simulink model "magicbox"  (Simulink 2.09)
settings: Solver=ode1  StartTime=0.0  StopTime=1  FixedStep=0.001  MaxStep=0.001  RelTol=1e-5  AbsTol=1e-6

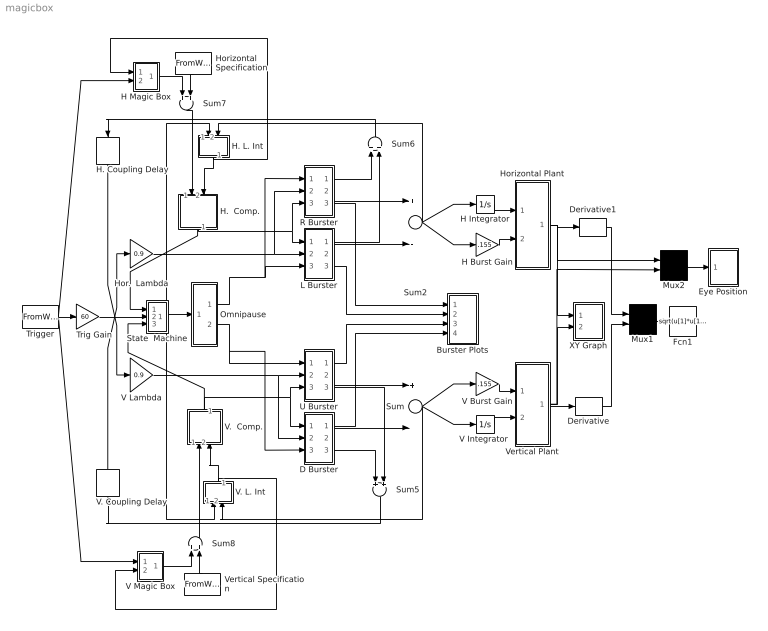
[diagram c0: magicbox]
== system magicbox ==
  Burster Plots : Subsystem
  D Burster : Subsystem
  Derivative : Derivative
  Derivative1 : Derivative
  Eye Position : Subsystem  mask(Graph scope.){}
      mask help: Graph scope using MATLAB graph window. Enter plotting ranges and line type.
      mask init:
      | color = @4; ax = [0, @1, @2, @3]; dt = -1;
  Fcn1 : Fcn  Expr=sqrt(u[1]*u[1]+u[2]*u[2])
  H Burst Gain : Gain  Gain=.155
  H Integrator : Integrator  ExternalReset=none  InitialConditionSource=internal  InitialCondition=0  LimitOutput=off  UpperSaturationLimit=inf  LowerSaturationLimit=-inf  ShowSaturationPort=off  ShowStatePort=off  AbsoluteTolerance=auto
  H Magic Box : Subsystem
  H.  Comp. : Subsystem  Orientation=down
  H. Coupling Delay : TransportDelay  Orientation=down  DelayTime=.001  InitialInput=00  BufferSize=1024
  H. L. Int : Subsystem  Orientation=down
  Hor.  Lambda : Gain  Gain=0.9
  Horizontal Plant : Subsystem
  "Horizontal Specification " : FromWorkspace  Orientation=down  VariableName=hspec
  L Burster : Subsystem
  Mux1 : Mux  Inputs=2
  Mux2 : Mux  Inputs=2
  Omnipause : Subsystem
  R Burster : Subsystem
  State  Machine : Subsystem
  Sum : Sum  Inputs=+-
  Sum2 : Sum  Inputs=+-
  Sum5 : Sum  Orientation=down  Inputs=++
  Sum6 : Sum  Orientation=up  Inputs=++
  Sum7 : Sum  Orientation=down  Inputs=++
  Sum8 : Sum  Orientation=up  Inputs=++
  Trig Gain : Gain  Gain=60
  Trigger : FromWorkspace  VariableName=trigspec
  U Burster : Subsystem
  V Burst Gain : Gain  Gain=.155
  "V Integrator " : Integrator  ExternalReset=none  InitialConditionSource=internal  InitialCondition=0  LimitOutput=off  UpperSaturationLimit=inf  LowerSaturationLimit=-inf  ShowSaturationPort=off  ShowStatePort=off  AbsoluteTolerance=auto
  V Lambda : Gain  Gain=0.9
  V Magic Box : Subsystem
  V.  Comp. : Subsystem  Orientation=up
  V. Coupling Delay : TransportDelay  Orientation=up  DelayTime=.001  InitialInput=00  BufferSize=1024
  V. L. Int : Subsystem  Orientation=up
  Vertical Plant : Subsystem
  Vertical Specification : FromWorkspace  Orientation=up  VariableName=vspec
  XY Graph : Subsystem  mask(XY scope.){}
      mask help: XY scope using MATLAB graph window. First input is used as time base. Enter plotting ranges.
      mask init:
      | ax = [@1, @2, @3, @4];st=-1;
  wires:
  H Integrator/1 -> Horizontal Plant/1(in_1)
  H Burst Gain/1 -> Horizontal Plant/2(in_2)
  Sum2/1 -> H Integrator/1, H Burst Gain/1, H. L. Int/2(BURST Input)
  V Burst Gain/1 -> Vertical Plant/1(in_1)
  "V Integrator "/1 -> Vertical Plant/2(in_2)
  Sum/1 -> V Burst Gain/1, "V Integrator "/1, V. L. Int/2(BURST Input)
  L Burster/2(out_2) -> Sum2/2
  R Burster/2(out_3) -> Sum2/1
  U Burster/3(out_4) -> Sum5/2
  U Burster/2(out_3) -> Sum/1
  U Burster/1(out_2) -> Burster Plots/3(in_3)
  D Burster/3(out_3) -> Sum5/1
  D Burster/2(out_2) -> Sum/2
  D Burster/1(out_1) -> Burster Plots/4(in_4)
  L Burster/3(out_3) -> Burster Plots/2(in_2)
  R Burster/3(out_4) -> Burster Plots/1(in_1)
  V Lambda/1 -> U Burster/2(in_2), D Burster/2(in_2)
  L Burster/1(out_1) -> Sum6/2
  Sum6/1 -> H. Coupling Delay/1
  Sum5/1 -> V. Coupling Delay/1
  Vertical Plant/1(out_1) -> XY Graph/2(y), Derivative/1, Mux2/2
  Mux1/1 -> Fcn1/1
  Derivative/1 -> Mux1/2
  Derivative1/1 -> Mux1/1
  Fcn1/1 -> ?
  R Burster/1(out_2) -> Sum6/1
  V. Coupling Delay/1 -> Hor.  Lambda/1
  H. Coupling Delay/1 -> V Lambda/1
  Horizontal Plant/1(out_1) -> XY Graph/1(x), Derivative1/1, Mux2/1
  Mux2/1 -> Eye Position/1(x)
  Hor.  Lambda/1 -> L Burster/2(in_2), R Burster/2(in_2)
  Omnipause/1(out_1) -> L Burster/3(in_3), R Burster/1(in_3)
  Omnipause/2(out_4) -> D Burster/3(in_3), U Burster/1(in_3)
  H.  Comp./1(out_1) -> L Burster/1(in_1), R Burster/3(in_1), State  Machine/1(in_1)
  V.  Comp./1(out_1) -> U Burster/3(in_1), D Burster/1(in_1), State  Machine/3(in_3)
  Trig Gain/1 -> State  Machine/2(in_2)
  State  Machine/1(out_2) -> V. L. Int/1(OPN Input), Omnipause/1(in_1), H. L. Int/1(STATE Input)
  "Horizontal Specification "/1 -> Sum7/2
  H Magic Box/1(out_1) -> Sum7/1
  Sum7/1 -> H.  Comp./1(in_1)
  H. L. Int/1(out_1) -> H.  Comp./2(in_2), H Magic Box/1(Current Displacement)
  Sum8/1 -> V.  Comp./1(in_4)
  Vertical Specification/1 -> Sum8/2
  V Magic Box/1(out_1) -> Sum8/1
  Trigger/1 -> Trig Gain/1, H Magic Box/2(Snapshot Trigger), V Magic Box/1(Current Displacement)
  V. L. Int/1(out_1) -> V.  Comp./2(in_5), V Magic Box/2(Snapshot Trigger)

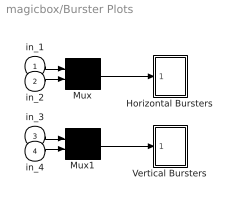
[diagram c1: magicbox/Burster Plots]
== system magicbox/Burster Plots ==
  in_1 : Inport  Port=1  PortWidth=-1  SampleTime=-1
  in_2 : Inport  Port=2  PortWidth=-1  SampleTime=-1
  in_3 : Inport  Port=3  PortWidth=-1  SampleTime=-1
  in_4 : Inport  Port=4  PortWidth=-1  SampleTime=-1
  Horizontal Bursters : Subsystem  mask(Graph scope.){}
      mask help: Graph scope using MATLAB graph window. Enter plotting ranges and line type.
      mask init:
      | color = @4; ax = [0, @1, @2, @3]; dt = -1;
  Mux : Mux  Inputs=2
  Mux1 : Mux  Inputs=2
  Vertical Bursters : Subsystem  mask(Graph scope.){}
      mask help: Graph scope using MATLAB graph window. Enter plotting ranges and line type.
      mask init:
      | color = @4; ax = [0, @1, @2, @3]; dt = -1;
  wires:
  Mux1/1 -> Vertical Bursters/1(x)
  Mux/1 -> Horizontal Bursters/1(x)
  in_1/1 -> Mux/1
  in_2/1 -> Mux/2
  in_3/1 -> Mux1/1
  in_4/1 -> Mux1/2

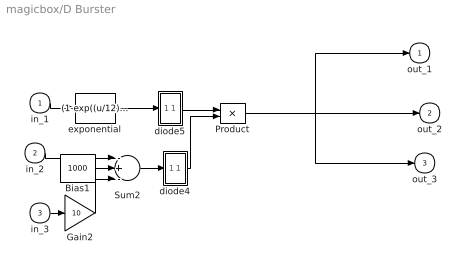
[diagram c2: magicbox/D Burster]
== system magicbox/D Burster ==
  in_1 : Inport  Port=1  PortWidth=-1  SampleTime=-1
  in_2 : Inport  Port=2  PortWidth=-1  SampleTime=-1
  in_3 : Inport  Port=3  PortWidth=-1  SampleTime=-1
  Bias1 : Constant  Value=1000
  Gain2 : Gain  Gain=10
  Product : Product  Inputs=2
  Sum2 : Sum  Inputs=-+-
  diode4 : Subsystem
  diode5 : Subsystem
  exponential : Fcn  Expr=(1-exp((u/12)))
  out_1 : Outport  Port=1  InitialOutput=0
  out_2 : Outport  Port=2  InitialOutput=0
  out_3 : Outport  Port=3  InitialOutput=0
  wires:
  Product/1 -> out_3/1, out_2/1, out_1/1
  diode5/1(out_1) -> Product/1
  exponential/1 -> diode5/1(in_1)
  diode4/1(out_1) -> Product/2
  Sum2/1 -> diode4/1(in_1)
  Gain2/1 -> Sum2/3
  in_3/1 -> Gain2/1
  in_2/1 -> Sum2/1
  Bias1/1 -> Sum2/2
  in_1/1 -> exponential/1

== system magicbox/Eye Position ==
  x : Inport  Port=1  PortWidth=-1  SampleTime=-1
  "S-function M-file which plots lines " : S-Function  FunctionName=sfuny  Parameters=ax, color,dt
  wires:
  x/1 -> "S-function M-file which plots lines "/1

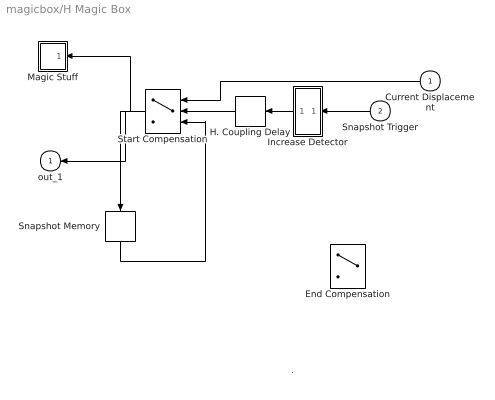
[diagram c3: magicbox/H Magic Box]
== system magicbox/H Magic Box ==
  note: .
  Current Displacement : Inport  Orientation=left  Port=1  PortWidth=-1  SampleTime=-1
  Snapshot Trigger : Inport  Orientation=left  Port=2  PortWidth=-1  SampleTime=-1
  " Snapshot Memory" : Memory  Orientation=down  X0=0  InheritSampleTime=off
  End Compensation : Switch  Orientation=left  Threshold=-2
  H. Coupling Delay : TransportDelay  Orientation=left  DelayTime=.002  InitialInput=00  BufferSize=1024
  Increase Detector : Subsystem  Orientation=left
  Magic Stuff : Subsystem  Orientation=left  mask(Graph scope.){}
      mask help: Graph scope using MATLAB graph window. Enter plotting ranges and line type.
      mask init:
      | color = @4; ax = [0, @1, @2, @3]; dt = -1;
  Start Compensation : Switch  Orientation=left  Threshold=0.001
  out_1 : Outport  Orientation=left  Port=1  InitialOutput=0
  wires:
  " Snapshot Memory"/1 -> Start Compensation/3
  Current Displacement/1 -> Start Compensation/1
  Start Compensation/1 -> " Snapshot Memory"/1, out_1/1, Magic Stuff/1(x)
  Snapshot Trigger/1 -> Increase Detector/1(Signal)
  Increase Detector/1(out_1) -> H. Coupling Delay/1
  H. Coupling Delay/1 -> Start Compensation/2

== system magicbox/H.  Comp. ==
  in_1 : Inport  Port=1  PortWidth=-1  SampleTime=-1
  in_2 : Inport  Port=2  PortWidth=-1  SampleTime=-1
  Sum : Sum  Inputs=+-
  out_1 : Outport  Port=1  InitialOutput=0
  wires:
  Sum/1 -> out_1/1
  in_1/1 -> Sum/1
  in_2/1 -> Sum/2

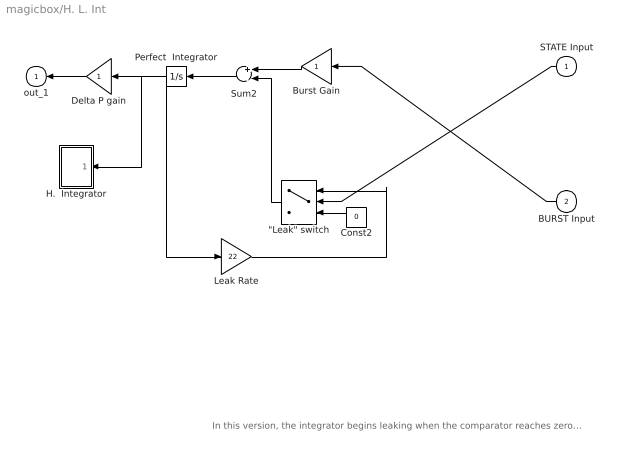
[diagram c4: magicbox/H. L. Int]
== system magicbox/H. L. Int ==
  note: In this version, the integrator begins leaking when the comparator reaches zero, and won't stop leaking until either the trigger arrives or the integrator's value goes to zero
  STATE Input : Inport  Orientation=left  Port=1  PortWidth=-1  SampleTime=-1
  BURST Input : Inport  Orientation=left  Port=2  PortWidth=-1  SampleTime=-1
  "\"Leak\" switch" : Switch  Orientation=left  Threshold=0.5
  Burst Gain : Gain  Orientation=left  Gain=1
  Const2 : Constant  Orientation=left  Value=0
  Delta P gain : Gain  Orientation=left  Gain=1
  H.  Integrator : Subsystem  Orientation=left  mask(Graph scope.){}
      mask help: Graph scope using MATLAB graph window. Enter plotting ranges and line type.
      mask init:
      | color = @4; ax = [0, @1, @2, @3]; dt = -1;
  Leak Rate : Gain  Gain=22
  Perfect  Integrator : Integrator  Orientation=left  ExternalReset=none  InitialConditionSource=internal  InitialCondition=0  LimitOutput=off  UpperSaturationLimit=inf  LowerSaturationLimit=-inf  ShowSaturationPort=off  ShowStatePort=off  AbsoluteTolerance=auto
  Sum2 : Sum  Orientation=left  Inputs=+-
  out_1 : Outport  Orientation=left  Port=1  InitialOutput=0
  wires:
  Sum2/1 -> Perfect  Integrator/1
  Delta P gain/1 -> out_1/1
  Burst Gain/1 -> Sum2/1
  Perfect  Integrator/1 -> Delta P gain/1, Leak Rate/1, H.  Integrator/1(x)
  Leak Rate/1 -> "\"Leak\" switch"/1
  "\"Leak\" switch"/1 -> Sum2/2
  Const2/1 -> "\"Leak\" switch"/3
  STATE Input/1 -> "\"Leak\" switch"/2
  BURST Input/1 -> Burst Gain/1

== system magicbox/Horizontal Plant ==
  in_1 : Inport  Orientation=left  Port=1  PortWidth=-1  SampleTime=-1
  in_2 : Inport  Orientation=left  Port=2  PortWidth=-1  SampleTime=-1
  Transfer Fcn1 : TransferFcn  Orientation=left  Numerator=[1]  Denominator=[.0018 .162 1]
  to Plant : Sum  Orientation=left  Inputs=++
  out_1 : Outport  Orientation=left  Port=1  InitialOutput=0
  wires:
  to Plant/1 -> Transfer Fcn1/1
  in_1/1 -> to Plant/1
  in_2/1 -> to Plant/2
  Transfer Fcn1/1 -> out_1/1

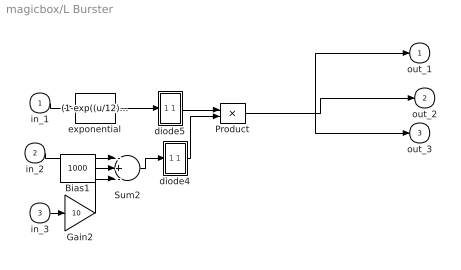
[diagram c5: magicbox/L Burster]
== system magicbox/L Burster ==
  in_1 : Inport  Port=1  PortWidth=-1  SampleTime=-1
  in_2 : Inport  Port=2  PortWidth=-1  SampleTime=-1
  in_3 : Inport  Port=3  PortWidth=-1  SampleTime=-1
  Bias1 : Constant  Value=1000
  Gain2 : Gain  Gain=10
  Product : Product  Inputs=2
  Sum2 : Sum  Inputs=-+-
  diode4 : Subsystem
  diode5 : Subsystem
  exponential : Fcn  Expr=(1-exp((u/12)))
  out_1 : Outport  Port=1  InitialOutput=0
  out_2 : Outport  Port=2  InitialOutput=0
  out_3 : Outport  Port=3  InitialOutput=0
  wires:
  in_1/1 -> exponential/1
  Bias1/1 -> Sum2/2
  in_2/1 -> Sum2/1
  in_3/1 -> Gain2/1
  Gain2/1 -> Sum2/3
  Sum2/1 -> diode4/1(in_1)
  diode4/1(out_1) -> Product/2
  exponential/1 -> diode5/1(in_1)
  diode5/1(out_1) -> Product/1
  Product/1 -> out_1/1, out_2/1, out_3/1

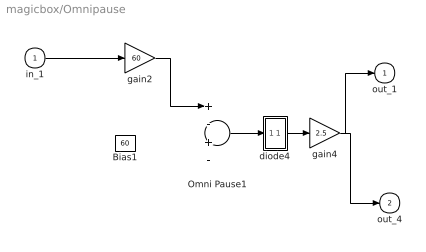
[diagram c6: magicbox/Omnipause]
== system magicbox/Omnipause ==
  in_1 : Inport  Port=1  PortWidth=-1  SampleTime=-1
  Bias1 : Constant  Value=60
  Omni Pause1 : Sum  Inputs=+-+-
  diode4 : Subsystem
  gain2 : Gain  Gain=60
  gain4 : Gain  Gain=2.5
  out_1 : Outport  Port=1  InitialOutput=0
  out_4 : Outport  Port=2  InitialOutput=0
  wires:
  Omni Pause1/1 -> diode4/1(in_1)
  ? -> Omni Pause1/2
  gain2/1 -> Omni Pause1/1
  diode4/1(out_1) -> gain4/1
  gain4/1 -> out_1/1, out_4/1
  in_1/1 -> gain2/1

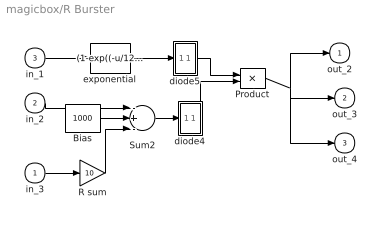
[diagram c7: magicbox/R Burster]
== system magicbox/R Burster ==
  in_3 : Inport  Port=1  PortWidth=-1  SampleTime=-1
  in_2 : Inport  Port=2  PortWidth=-1  SampleTime=-1
  in_1 : Inport  Port=3  PortWidth=-1  SampleTime=-1
  Bias : Constant  Value=1000
  Product : Product  Inputs=2
  R sum : Gain  Gain=10
  Sum2 : Sum  Inputs=-+-
  diode4 : Subsystem
  diode5 : Subsystem
  exponential : Fcn  Expr=(1-exp((-u/12)))
  out_2 : Outport  Port=1  InitialOutput=0
  out_3 : Outport  Port=2  InitialOutput=0
  out_4 : Outport  Port=3  InitialOutput=0
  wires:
  R sum/1 -> Sum2/3
  in_3/1 -> R sum/1
  Product/1 -> out_3/1, out_4/1, out_2/1
  Bias/1 -> Sum2/2
  in_2/1 -> Sum2/1
  in_1/1 -> exponential/1
  Sum2/1 -> diode4/1(in_1)
  diode4/1(out_1) -> Product/2
  exponential/1 -> diode5/1(in_1)
  diode5/1(out_1) -> Product/1

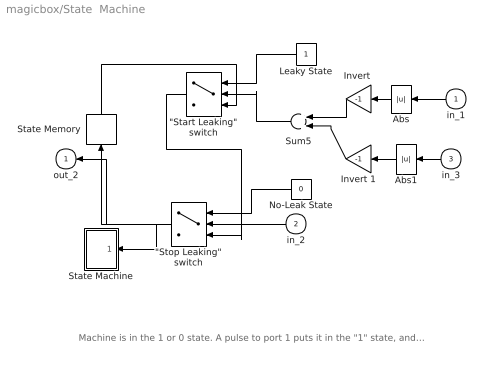
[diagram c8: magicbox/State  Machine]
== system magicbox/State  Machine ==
  note: Machine is in the 1 or 0 state. A pulse to port 1 puts it in the "1" state, and a pulse to port 2 puts it in the "0" state.
  in_1 : Inport  Orientation=left  Port=1  PortWidth=-1  SampleTime=-1
  in_2 : Inport  Orientation=left  Port=2  PortWidth=-1  SampleTime=-1
  in_3 : Inport  Orientation=left  Port=3  PortWidth=-1  SampleTime=-1
  "\"Start Leaking\" switch" : Switch  Orientation=left  Threshold=-2
  "\"Stop Leaking\" switch" : Switch  Orientation=left  Threshold=0.001
  Abs : Abs  Orientation=left
  Abs1 : Abs  Orientation=left
  "Invert " : Gain  Orientation=left  Gain=-1
  Invert 1 : Gain  Orientation=left  Gain=-1
  Leaky State : Constant  Orientation=left  Value=1
  No-Leak State : Constant  Orientation=left  Value=0
  State Memory : Memory  Orientation=up  X0=0  InheritSampleTime=off
  State Machine : Subsystem  Orientation=left  mask(Graph scope.){}
      mask help: Graph scope using MATLAB graph window. Enter plotting ranges and line type.
      mask init:
      | color = @4; ax = [0, @1, @2, @3]; dt = -1;
  Sum5 : Sum  Orientation=left  Inputs=++
  out_2 : Outport  Orientation=left  Port=1  InitialOutput=0
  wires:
  in_2/1 -> "\"Stop Leaking\" switch"/2
  in_1/1 -> Abs/1
  "\"Stop Leaking\" switch"/1 -> out_2/1, State Memory/1, State Machine/1(x)
  Abs/1 -> "Invert "/1
  State Memory/1 -> "\"Start Leaking\" switch"/3
  Leaky State/1 -> "\"Start Leaking\" switch"/1
  "\"Start Leaking\" switch"/1 -> "\"Stop Leaking\" switch"/3
  No-Leak State/1 -> "\"Stop Leaking\" switch"/1
  in_3/1 -> Abs1/1
  Abs1/1 -> Invert 1/1
  Invert 1/1 -> Sum5/2
  "Invert "/1 -> Sum5/1
  Sum5/1 -> "\"Start Leaking\" switch"/2

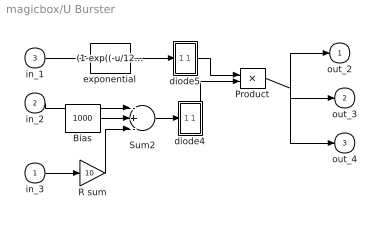
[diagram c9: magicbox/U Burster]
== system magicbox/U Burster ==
  in_3 : Inport  Port=1  PortWidth=-1  SampleTime=-1
  in_2 : Inport  Port=2  PortWidth=-1  SampleTime=-1
  in_1 : Inport  Port=3  PortWidth=-1  SampleTime=-1
  Bias : Constant  Value=1000
  Product : Product  Inputs=2
  R sum : Gain  Gain=10
  Sum2 : Sum  Inputs=-+-
  diode4 : Subsystem
  diode5 : Subsystem
  exponential : Fcn  Expr=(1-exp((-u/12)))
  out_2 : Outport  Port=1  InitialOutput=0
  out_3 : Outport  Port=2  InitialOutput=0
  out_4 : Outport  Port=3  InitialOutput=0
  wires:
  R sum/1 -> Sum2/3
  in_3/1 -> R sum/1
  Product/1 -> out_3/1, out_4/1, out_2/1
  Bias/1 -> Sum2/2
  in_2/1 -> Sum2/1
  in_1/1 -> exponential/1
  Sum2/1 -> diode4/1(in_1)
  diode4/1(out_1) -> Product/2
  exponential/1 -> diode5/1(in_1)
  diode5/1(out_1) -> Product/1

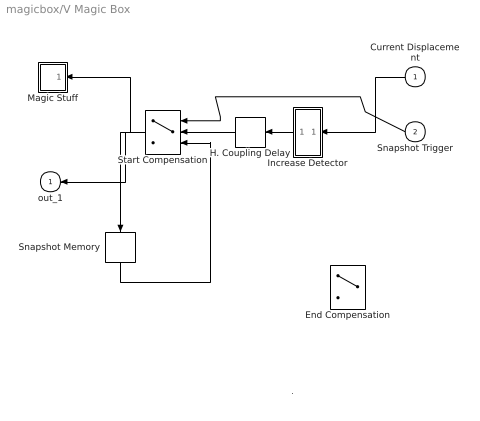
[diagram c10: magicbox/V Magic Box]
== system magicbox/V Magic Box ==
  note: .
  Current Displacement : Inport  Orientation=left  Port=1  PortWidth=-1  SampleTime=-1
  Snapshot Trigger : Inport  Orientation=left  Port=2  PortWidth=-1  SampleTime=-1
  " Snapshot Memory" : Memory  Orientation=down  X0=0  InheritSampleTime=off
  End Compensation : Switch  Orientation=left  Threshold=-2
  H. Coupling Delay : TransportDelay  Orientation=left  DelayTime=.002  InitialInput=00  BufferSize=1024
  Increase Detector : Subsystem  Orientation=left
  Magic Stuff : Subsystem  Orientation=left  mask(Graph scope.){}
      mask help: Graph scope using MATLAB graph window. Enter plotting ranges and line type.
      mask init:
      | color = @4; ax = [0, @1, @2, @3]; dt = -1;
  Start Compensation : Switch  Orientation=left  Threshold=0.001
  out_1 : Outport  Orientation=left  Port=1  InitialOutput=0
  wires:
  " Snapshot Memory"/1 -> Start Compensation/3
  Start Compensation/1 -> " Snapshot Memory"/1, out_1/1, Magic Stuff/1(x)
  Increase Detector/1(out_1) -> H. Coupling Delay/1
  H. Coupling Delay/1 -> Start Compensation/2
  Current Displacement/1 -> Increase Detector/1(Signal)
  Snapshot Trigger/1 -> Start Compensation/1

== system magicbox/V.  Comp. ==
  in_4 : Inport  Port=1  PortWidth=-1  SampleTime=-1
  in_5 : Inport  Port=2  PortWidth=-1  SampleTime=-1
  Sum : Sum  Inputs=-+
  out_1 : Outport  Port=1  InitialOutput=0
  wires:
  Sum/1 -> out_1/1
  in_5/1 -> Sum/1
  in_4/1 -> Sum/2

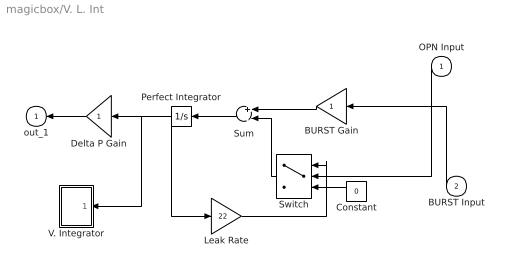
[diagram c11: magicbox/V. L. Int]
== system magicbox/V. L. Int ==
  OPN Input : Inport  Orientation=left  Port=1  PortWidth=-1  SampleTime=-1
  BURST Input : Inport  Orientation=left  Port=2  PortWidth=-1  SampleTime=-1
  BURST Gain : Gain  Orientation=left  Gain=1
  Constant : Constant  Orientation=left  Value=0
  Delta P Gain : Gain  Orientation=left  Gain=1
  Leak Rate : Gain  Gain=22
  Perfect Integrator : Integrator  Orientation=left  ExternalReset=none  InitialConditionSource=internal  InitialCondition=0  LimitOutput=off  UpperSaturationLimit=inf  LowerSaturationLimit=-inf  ShowSaturationPort=off  ShowStatePort=off  AbsoluteTolerance=auto
  Sum : Sum  Orientation=left  Inputs=+-
  Switch : Switch  Orientation=left  Threshold=0.5
  V. Integrator : Subsystem  Orientation=left  mask(Graph scope.){}
      mask help: Graph scope using MATLAB graph window. Enter plotting ranges and line type.
      mask init:
      | color = @4; ax = [0, @1, @2, @3]; dt = -1;
  out_1 : Outport  Orientation=left  Port=1  InitialOutput=0
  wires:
  Switch/1 -> Sum/2
  Constant/1 -> Switch/3
  Leak Rate/1 -> Switch/1
  Perfect Integrator/1 -> V. Integrator/1(x), Leak Rate/1, Delta P Gain/1
  BURST Gain/1 -> Sum/1
  Delta P Gain/1 -> out_1/1
  Sum/1 -> Perfect Integrator/1
  OPN Input/1 -> Switch/2
  BURST Input/1 -> BURST Gain/1

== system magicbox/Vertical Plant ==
  in_1 : Inport  Orientation=left  Port=1  PortWidth=-1  SampleTime=-1
  in_2 : Inport  Orientation=left  Port=2  PortWidth=-1  SampleTime=-1
  Transfer Fcn1 : TransferFcn  Orientation=left  Numerator=[1]  Denominator=[.0018 .162 1]
  to Plant : Sum  Orientation=left  Inputs=++
  out_1 : Outport  Orientation=left  Port=1  InitialOutput=0
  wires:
  to Plant/1 -> Transfer Fcn1/1
  in_1/1 -> to Plant/1
  in_2/1 -> to Plant/2
  Transfer Fcn1/1 -> out_1/1

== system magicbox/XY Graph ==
  x : Inport  Port=1  PortWidth=-1  SampleTime=-1
  y : Inport  Port=2  PortWidth=-1  SampleTime=-1
  Mux : Mux  Inputs=2
  "S-function M-file which plots lines " : S-Function  FunctionName=sfunxy  Parameters=ax, st
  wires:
  y/1 -> Mux/2
  x/1 -> Mux/1
  Mux/1 -> "S-function M-file which plots lines "/1

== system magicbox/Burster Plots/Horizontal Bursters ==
  x : Inport  Port=1  PortWidth=-1  SampleTime=-1
  "S-function M-file which plots lines " : S-Function  FunctionName=sfuny  Parameters=ax, color,dt
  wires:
  x/1 -> "S-function M-file which plots lines "/1

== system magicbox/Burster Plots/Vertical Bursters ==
  x : Inport  Port=1  PortWidth=-1  SampleTime=-1
  "S-function M-file which plots lines " : S-Function  FunctionName=sfuny  Parameters=ax, color,dt
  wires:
  x/1 -> "S-function M-file which plots lines "/1

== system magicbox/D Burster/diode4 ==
  in_1 : Inport  Port=1  PortWidth=-1  SampleTime=-1
  Switch : Switch  Threshold=0
  diode1 : Constant  Value=0
  out_1 : Outport  Port=1  InitialOutput=0
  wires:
  diode1/1 -> Switch/3
  Switch/1 -> out_1/1
  in_1/1 -> Switch/1, Switch/2

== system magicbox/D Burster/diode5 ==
  in_1 : Inport  Port=1  PortWidth=-1  SampleTime=-1
  Switch : Switch  Threshold=0
  diode1 : Constant  Value=0
  out_1 : Outport  Port=1  InitialOutput=0
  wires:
  diode1/1 -> Switch/3
  Switch/1 -> out_1/1
  in_1/1 -> Switch/1, Switch/2

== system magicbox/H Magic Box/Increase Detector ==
  note: Increase Detector compares Signal at time t to signal at time t-1. When difference is greater than the Switch threshold, it outputs the difference (positive), 0 otherwise.
  Signal : Inport  Port=1  PortWidth=-1  SampleTime=-1
  Memory : Memory  X0=0  InheritSampleTime=off
  Sum6 : Sum  Inputs=+-
  Switch : Switch  Threshold=0.001
  This output means no detection : Constant  Value=0
  out_1 : Outport  Port=1  InitialOutput=0
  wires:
  Switch/1 -> out_1/1
  Signal/1 -> Sum6/1, Memory/1
  Memory/1 -> Sum6/2
  Sum6/1 -> Switch/2, Switch/1
  This output means no detection/1 -> Switch/3

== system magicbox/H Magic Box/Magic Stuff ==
  x : Inport  Port=1  PortWidth=-1  SampleTime=-1
  "S-function M-file which plots lines " : S-Function  FunctionName=sfuny  Parameters=ax, color,dt
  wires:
  x/1 -> "S-function M-file which plots lines "/1

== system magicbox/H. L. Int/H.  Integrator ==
  x : Inport  Port=1  PortWidth=-1  SampleTime=-1
  "S-function M-file which plots lines " : S-Function  FunctionName=sfuny  Parameters=ax, color,dt
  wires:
  x/1 -> "S-function M-file which plots lines "/1

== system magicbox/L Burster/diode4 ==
  in_1 : Inport  Port=1  PortWidth=-1  SampleTime=-1
  Switch : Switch  Threshold=0
  diode1 : Constant  Value=0
  out_1 : Outport  Port=1  InitialOutput=0
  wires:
  in_1/1 -> Switch/1, Switch/2
  Switch/1 -> out_1/1
  diode1/1 -> Switch/3

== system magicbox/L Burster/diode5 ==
  in_1 : Inport  Port=1  PortWidth=-1  SampleTime=-1
  Switch : Switch  Threshold=0
  diode1 : Constant  Value=0
  out_1 : Outport  Port=1  InitialOutput=0
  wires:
  in_1/1 -> Switch/1, Switch/2
  Switch/1 -> out_1/1
  diode1/1 -> Switch/3

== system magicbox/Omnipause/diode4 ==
  in_1 : Inport  Port=1  PortWidth=-1  SampleTime=-1
  Switch : Switch  Threshold=0
  diode1 : Constant  Value=0
  out_1 : Outport  Port=1  InitialOutput=0
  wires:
  diode1/1 -> Switch/3
  Switch/1 -> out_1/1
  in_1/1 -> Switch/1, Switch/2

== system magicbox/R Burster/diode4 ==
  in_1 : Inport  Port=1  PortWidth=-1  SampleTime=-1
  Switch : Switch  Threshold=0
  diode1 : Constant  Value=0
  out_1 : Outport  Port=1  InitialOutput=0
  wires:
  diode1/1 -> Switch/3
  Switch/1 -> out_1/1
  in_1/1 -> Switch/1, Switch/2

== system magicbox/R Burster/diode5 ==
  in_1 : Inport  Port=1  PortWidth=-1  SampleTime=-1
  Switch : Switch  Threshold=0
  diode1 : Constant  Value=0
  out_1 : Outport  Port=1  InitialOutput=0
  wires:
  in_1/1 -> Switch/1, Switch/2
  Switch/1 -> out_1/1
  diode1/1 -> Switch/3

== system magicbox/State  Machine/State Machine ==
  x : Inport  Port=1  PortWidth=-1  SampleTime=-1
  "S-function M-file which plots lines " : S-Function  FunctionName=sfuny  Parameters=ax, color,dt
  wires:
  x/1 -> "S-function M-file which plots lines "/1

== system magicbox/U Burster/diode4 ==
  in_1 : Inport  Port=1  PortWidth=-1  SampleTime=-1
  Switch : Switch  Threshold=0
  diode1 : Constant  Value=0
  out_1 : Outport  Port=1  InitialOutput=0
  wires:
  diode1/1 -> Switch/3
  Switch/1 -> out_1/1
  in_1/1 -> Switch/1, Switch/2

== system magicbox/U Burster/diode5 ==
  in_1 : Inport  Port=1  PortWidth=-1  SampleTime=-1
  Switch : Switch  Threshold=0
  diode1 : Constant  Value=0
  out_1 : Outport  Port=1  InitialOutput=0
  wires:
  in_1/1 -> Switch/1, Switch/2
  Switch/1 -> out_1/1
  diode1/1 -> Switch/3

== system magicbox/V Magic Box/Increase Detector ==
  note: Increase Detector compares Signal at time t to signal at time t-1. When difference is greater than the Switch threshold, it outputs the difference (positive), 0 otherwise.
  Signal : Inport  Port=1  PortWidth=-1  SampleTime=-1
  Memory : Memory  X0=0  InheritSampleTime=off
  Sum6 : Sum  Inputs=+-
  Switch : Switch  Threshold=0.001
  This output means no detection : Constant  Value=0
  out_1 : Outport  Port=1  InitialOutput=0
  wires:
  Switch/1 -> out_1/1
  Signal/1 -> Sum6/1, Memory/1
  Memory/1 -> Sum6/2
  Sum6/1 -> Switch/2, Switch/1
  This output means no detection/1 -> Switch/3

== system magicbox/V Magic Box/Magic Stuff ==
  x : Inport  Port=1  PortWidth=-1  SampleTime=-1
  "S-function M-file which plots lines " : S-Function  FunctionName=sfuny  Parameters=ax, color,dt
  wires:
  x/1 -> "S-function M-file which plots lines "/1

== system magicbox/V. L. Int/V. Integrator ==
  x : Inport  Port=1  PortWidth=-1  SampleTime=-1
  "S-function M-file which plots lines " : S-Function  FunctionName=sfuny  Parameters=ax, color,dt
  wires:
  x/1 -> "S-function M-file which plots lines "/1
